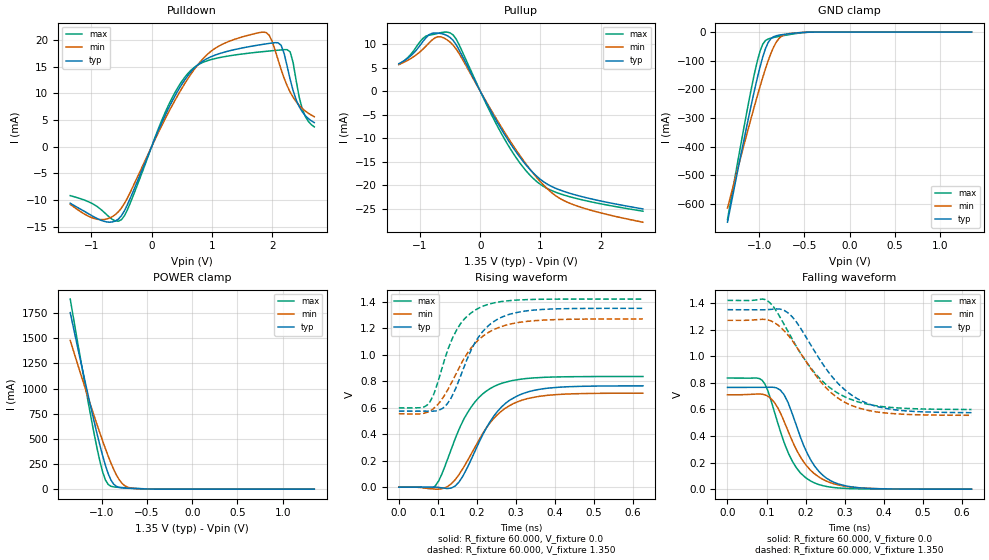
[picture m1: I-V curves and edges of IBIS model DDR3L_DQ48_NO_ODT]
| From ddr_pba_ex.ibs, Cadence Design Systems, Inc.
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|   Model DDR3L_DQ48_NO_ODT
[Model]   DDR3L_DQ48_NO_ODT
Model_type I/O
Polarity   Non-Inverting
Enable   Active-High
Vinl   =   0.624V
Vinh   =   0.727V
C_comp   1.704pF   1.694pF   1.708pF
C_comp_pullup   0.520pF   0.541pF   0.498pF
C_comp_pulldown 1.183pF   1.153pF   1.209pF
[Model Spec]
Vinh   0.727V   NA   NA
Vinl   0.624V   NA   NA
Vmeas   0.675V   NA   NA
[Temperature Range]   27.000   0.125k   -40.000
[Voltage Range]   1.350V   1.270V   1.420V
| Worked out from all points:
|   slope of the pulldown table from 0 to 0.203 V, typ, clamps not added: 38 ohm
|   slope of the pullup table from 0 to 0.203 V, typ, clamps not added: 41.9 ohm
|   GND clamp passes 1 mA (typ) near -0.50 V on its own axis
|   POWER clamp passes 1 mA (typ) near -0.46 V on its own axis
|   rising waveform, R_fixture 60.000, V_fixture 0.0: 20-80 % time 89ps typ, 95.7ps min, 83.1ps max; typ from 0 V to 0.765 V
|   rising waveform, R_fixture 60.000, V_fixture 1.350: 20-80 % time 77.7ps typ, 92.1ps min, 67.3ps max; typ from 0.575 V to 1.35 V
|   falling waveform, R_fixture 60.000, V_fixture 0.0: 20-80 % time 68.4ps typ, 76.7ps min, 63.7ps max; typ from 0.765 V to 0 V
|   falling waveform, R_fixture 60.000, V_fixture 1.350: 20-80 % time 117ps typ, 113ps min, 120ps max; typ from 1.35 V to 0.576 V
[Pulldown]
|Voltage   I(typ)   I(min)   I(max)
-1.35V    -10.59mA   -10.79mA   -9.165mA
-850mV    -13.73mA   -13.67mA   -11.67mA
-500mV    -12.92mA   -11.5mA    -13.67mA
200mV     5.271mA    4.664mA    5.784mA
500mV     11.68mA    10.91mA    12.24mA
900mV     16.41mA    17.05mA    16.04mA
1.35V     18.15mA    20.04mA    17.16mA
1.95V     19.38mA    20.93mA    17.95mA
2.15V     19.02mA    14.47mA    18.16mA
2.3V      12.6mA     10.24mA    17.78mA
2.5V      6.561mA    7.181mA    7.107mA
2.7V      4.533mA    5.632mA    3.721mA
[Pullup]
|Voltage   I(typ)   I(min)   I(max)
-1.35V    5.83mA     5.65mA     5.655mA
-1.1V     8.144mA    7.344mA    8.639mA
-850mV    11.96mA    10.22mA    11.87mA
-700mV    12.33mA    11.56mA    12.27mA
-500mV    11.4mA     10.4mA     12.38mA
-350mV    8.759mA    7.978mA    9.845mA
400mV     -9.144mA   -8.667mA   -10.13mA
650mV     -13.91mA   -13.54mA   -15.14mA
900mV     -17.66mA   -17.81mA   -18.82mA
1.2V      -20.38mA   -21.75mA   -21.24mA
1.45V     -21.59mA   -23.66mA   -22.34mA
2.7V      -25.07mA   -27.88mA   -25.55mA
[GND_clamp]
|Voltage   I(typ)   I(min)   I(max)
-1.35V    -663.5mA   -614.2mA   -654.4mA
-1.17V    -379.6mA   -396.8mA   -336.4mA
-1.05V    -201.2mA   -256.6mA   -142.3mA
-990mV    -121.8mA   -190.1mA   -66.76mA
-960mV    -87.12mA   -158.5mA   -42.47mA
-930mV    -58.01mA   -128.3mA   -29.57mA
-870mV    -23.03mA   -74.64mA   -21.11mA
-810mV    -12.75mA   -34.94mA   -17.06mA
-750mV    -9.218mA   -14.09mA   -13.42mA
-690mV    -6.687mA   -6.669mA   -9.983mA
-420mV    -175.8uA   -266.9uA   -234.9uA
1.35V     1.792nA    307.1nA    263.8pA
[POWER_clamp]
|Voltage   I(typ)   I(min)   I(max)
-1.35V    1.755A     1.479A     1.89A
-1.17V    1.006A     962.6mA    958.1mA
-1.05V    538.4mA    632.4mA    392.2mA
-990mV    328mA      475.7mA    167mA
-960mV    234.7mA    400.6mA    90.32mA
-930mV    154.2mA    328.7mA    47.17mA
-900mV    91.53mA    260.8mA    29.3mA
-870mV    50.28mA    198.1mA    22.68mA
-780mV    13.3mA     60.49mA    15.94mA
-720mV    9.309mA    21.57mA    12.7mA
-660mV    6.902mA    8.818mA    9.643mA
1.35V     -4.773nA   -193.5nA   -1.001nA
[Ramp]
| variable   typ   min   max
dV/dt_r 0.419/87.454p   0.390/93.373p   0.458/80.404p
dV/dt_f 0.420/0.116n   0.391/0.112n   0.440/0.119n
R_load = 50.000
| The next line is not an IBIS keyword
| [Initial Delay]   0.200ns   0.400ns   0.150ns
[Rising Waveform]
R_fixture= 60.000
V_fixture= 0.0
V_fixture_min= 0.0
V_fixture_max= 0.0
|time   V(typ)   V(min)   V(max)
0s        8.065uV    771.2uV    -12.06uV
90ps      1.491mV    -13.68mV   917.6uV
109ps     -4.526mV   -11.95mV   91.01mV
144ps     8.599mV    55.57mV    364.3mV
164ps     83.69mV    140.7mV    499.3mV
193ps     259.9mV    293.2mV    636.9mV
244ps     540.3mV    521.5mV    761.1mV
284ps     657.3mV    616.9mV    800.9mV
352ps     734.7mV    682.3mV    826.5mV
625ps     765mV      709.9mV    835.9mV
[Rising Waveform]
R_fixture= 60.000
V_fixture= 1.350
V_fixture_min= 1.270
V_fixture_max= 1.420
|time   V(typ)   V(min)   V(max)
0s        574.5mV    554.4mV    598.4mV
73ps      573.7mV    565.8mV    621.2mV
90ps      574.2mV    596.4mV    707mV
116ps     604.3mV    689.3mV    952.6mV
158ps     838.3mV    923.3mV    1.234V
184ps     1.029V     1.047V     1.313V
215ps     1.176V     1.14V      1.366V
263ps     1.283V     1.213V     1.402V
323ps     1.33V      1.25V      1.416V
625ps     1.35V      1.27V      1.42V
[Falling Waveform]
R_fixture= 60.000
V_fixture= 0.0
V_fixture_min= 0.0
V_fixture_max= 0.0
|time   V(typ)   V(min)   V(max)
0s        765.2mV    710mV      836mV
89ps      764.9mV    714.6mV    818.3mV
102ps     766.2mV    701.3mV    751.4mV
135ps     746.2mV    576.1mV    438.4mV
155ps     652.3mV    438.9mV    277.7mV
176ps     481.6mV    300.5mV    162.7mV
221ps     183.4mV    119.9mV    49.01mV
263ps     65.3mV     49.31mV    15.75mV
314ps     18.8mV     16.37mV    4.308mV
625ps     42.97uV    88.37uV    39.85uV
[Falling Waveform]
R_fixture= 60.000
V_fixture= 1.350
V_fixture_min= 1.270
V_fixture_max= 1.420
|time   V(typ)   V(min)   V(max)
0s        1.35V      1.27V      1.42V
102ps     1.35V      1.274V     1.418V
119ps     1.354V     1.255V     1.367V
155ps     1.326V     1.159V     1.186V
228ps     1.013V     847.6mV    859mV
265ps     856.5mV    726.3mV    757.3mV
308ps     729.2mV    641.9mV    684.6mV
353ps     650.9mV    597mV      642.5mV
413ps     603.6mV    570.6mV    616.1mV
625ps     575.5mV    555.6mV    599.2mV
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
